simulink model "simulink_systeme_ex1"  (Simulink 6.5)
settings: Solver=ode45  StartTime=0.0  StopTime=0.2  RelTol=1e-3
PostLoadFcn:
  | simulink_systems_ex1
StartFcn:
  | simulink_systems_ex1
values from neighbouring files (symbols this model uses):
  T1 = 0.01    [simulink_systems_ex1.m]
  V = 1    [simulink_systems_ex1.m]

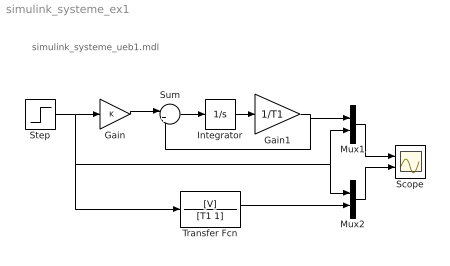
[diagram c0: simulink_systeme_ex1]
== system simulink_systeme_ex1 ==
  note: simulink_systeme_ueb1.mdl
  Gain : Gain
  Gain1 : Gain  Gain=1/T1
  Integrator : Integrator
  Mux1 : Mux  Inputs=2
  Mux2 : Mux  Inputs=2
  Scope : Scope  NumInputPorts=2
  Step : Step  Time=.1  SampleTime=0
  Sum : Sum  Inputs=|+-
  Transfer Fcn : TransferFcn  Numerator=[V]  Denominator=[T1 1]
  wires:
  Step/1 -> Gain/1, Transfer Fcn/1, Mux1/2, Mux2/1
  Gain/1 -> Sum/1
  Sum/1 -> Integrator/1
  Integrator/1 -> Gain1/1
  Gain1/1 -> Sum/2, Mux1/1
  Mux1/1 -> Scope/1
  Transfer Fcn/1 -> Mux2/2
  Mux2/1 -> Scope/2
